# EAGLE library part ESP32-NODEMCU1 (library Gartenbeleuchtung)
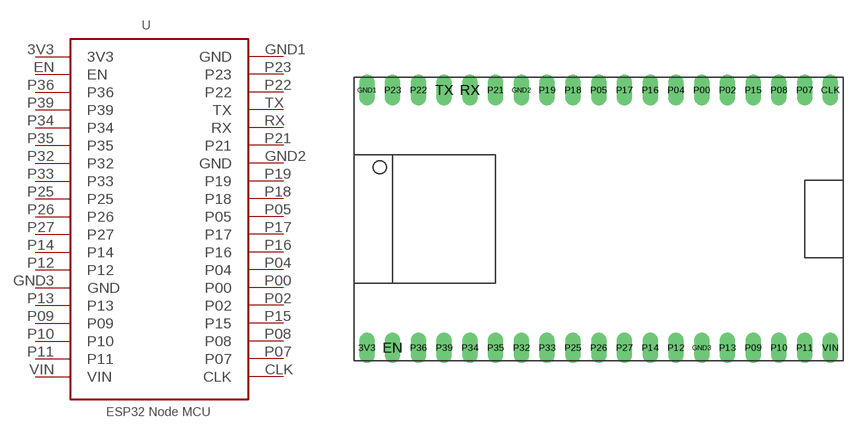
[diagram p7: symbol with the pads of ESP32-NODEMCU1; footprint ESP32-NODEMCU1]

Designator prefix -

## ESP32-NODEMCU1  [ESP32-NODEMCU1]
3V3  3V3  pwr
CLK  CLK
EN  EN
GND1  GND  pwr
GND2  GND  pwr
GND3  GND  pwr
P00  P00
P02  P02
P04  P04
P05  P05
P07  P07
P08  P08
P09  P09
P10  P10
P11  P11
P12  P12
P13  P13
P14  P14
P15  P15
P16  P16
P17  P17
P18  P18
P19  P19
P21  P21
P22  P22
P23  P23
P25  P25
P26  P26
P27  P27
P32  P32
P33  P33
P34  P34
P35  P35
P36  P36
P39  P39
RX  RX
TX  TX
VIN  VIN  pwr

## Footprint ESP32-NODEMCU1 (pad centres in mm)
drill 1 pad 1.422 long: 3V3 -22.86,-12.7; CLK 22.86,12.7; EN -20.32,-12.7; GND1 -22.86,12.7; GND2 -7.62,12.7; GND3 10.16,-12.7; P00 10.16,12.7; P02 12.7,12.7; P04 7.62,12.7; P05 0,12.7; P07 20.32,12.7; P08 17.78,12.7; P09 15.24,-12.7; P10 17.78,-12.7; P11 20.32,-12.7; P12 7.62,-12.7; P13 12.7,-12.7; P14 5.08,-12.7; P15 15.24,12.7; P16 5.08,12.7; P17 2.54,12.7; P18 -2.54,12.7; P19 -5.08,12.7; P21 -10.16,12.7; P22 -17.78,12.7; P23 -20.32,12.7; P25 -2.54,-12.7; P26 0,-12.7; P27 2.54,-12.7; P32 -7.62,-12.7; P33 -5.08,-12.7; P34 -12.7,-12.7; P35 -10.16,-12.7; P36 -17.78,-12.7; P39 -15.24,-12.7; RX -12.7,12.7; TX -15.24,12.7; VIN 22.86,-12.7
